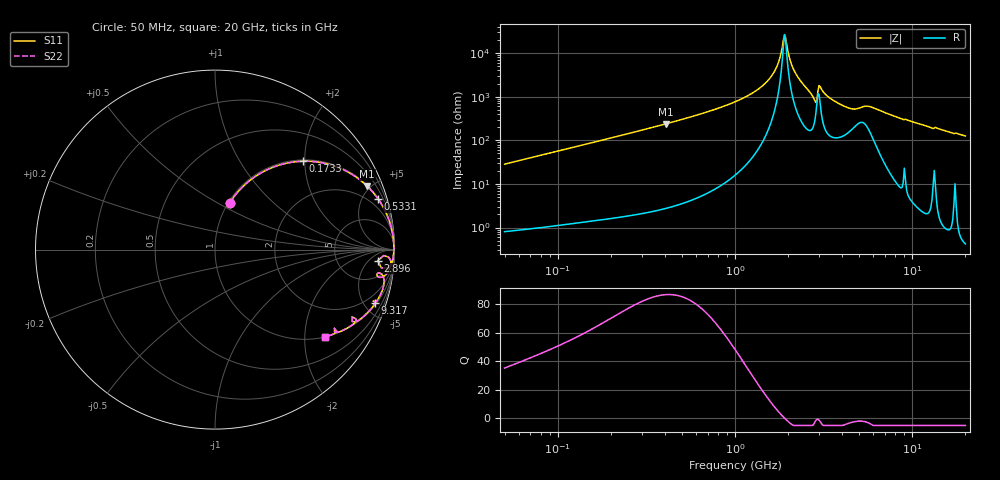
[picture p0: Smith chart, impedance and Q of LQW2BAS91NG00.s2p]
!Murata Part Number: LQW2BAS91NG00
!These Parameters are Measured in Series Mode Connection
!  o--[Z]--o
!Port1  Port2
!  o-------o
!Freq. Start=50[MHz] Stop=20[GHz], 401[Steps]
# Hz S RI R 50
!Freq.(Hz) S11(Real) S11(Imag) S21(Real) S21(Imag) S12(Real) S12(Imag) S22(Real) S22(Imag)
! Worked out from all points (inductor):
!   401 points, 50 MHz to 20 GHz, reference 50 ohm
!   read as one part in series: L = 90.2 nH near 51.52 MHz
!   highest Q = 86.9 at 407.1 MHz (marker M1), where L = 93.3 nH
!   self-resonance near 1.904 GHz
!   S11 on the Smith chart (normalised r, x): 50 MHz: 1.02, +0.57; 173.3 MHz: 1.03, +1.97; 533.1 MHz: 1.08, +6.46; 2.896 GHz: 14, -10; 9.317 GHz: 1.14, -5.91; 20 GHz: 1.01, -2.52
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5e7  0.081 0.2591  0.919 -0.2591  0.919 -0.2591  0.081 0.2591
1.364002e8  0.3756 0.4759  0.6244 -0.4759  0.6244 -0.4759  0.3756 0.4759
1.733395e8  0.4915 0.4924  0.5085 -0.4924  0.5085 -0.4924  0.4915 0.4924
3.721004e8  0.8214 0.3773  0.1786 -0.3773  0.1786 -0.3773  0.8214 0.3773
4.070905e8  0.8478 0.3535  0.1522 -0.3535  0.1522 -0.3535  0.8478 0.3535
5.330693e8  0.9098 0.2806  0.0902 -0.2806  0.0902 -0.2806  0.9098 0.2806
1e9  0.9806 0.1281  0.0194 -0.1281  0.0194 -0.1281  0.9806 0.1281
1.309461e9  0.9919 0.0728  0.00814 -0.0728  0.00814 -0.0728  0.9919 0.0728
1.567309e9  0.9955 0.038  0.00451 -0.038  0.00451 -0.038  0.9955 0.038
1.740566e9  0.9963 0.0179  0.00366 -0.0179  0.00366 -0.0179  0.9963 0.0179
1.904239e9  0.9963 0.000534  0.00369 -0.000534  0.00369 -0.000534  0.9963 0.000534
2.179053e9  0.9947 -0.0265  0.00529 0.0265  0.00529 0.0265  0.9947 -0.0265
2.728004e9  0.9764 -0.0887  0.0236 0.0887  0.0236 0.0887  0.9764 -0.0887
2.810964e9  0.9538 -0.1041  0.0462 0.1041  0.0462 0.1041  0.9538 -0.1041
2.896447e9  0.9078 -0.0609  0.0922 0.0609  0.0922 0.0609  0.9078 -0.0609
3.029571e9  0.9746 -0.0519  0.0254 0.0519  0.0254 0.0519  0.9746 -0.0519
3.415248e9  0.9753 -0.101  0.0247 0.101  0.0247 0.101  0.9753 -0.101
4.212059e9  0.9382 -0.1499  0.0618 0.1499  0.0618 0.1499  0.9382 -0.1499
5.598765e9  0.9288 -0.1376  0.0712 0.1376  0.0712 0.1376  0.9288 -0.1376
7.442007e9  0.9298 -0.233  0.0702 0.233  0.0702 0.233  0.9298 -0.233
9.316812e9  0.8917 -0.2989  0.1083 0.2989  0.1083 0.2989  0.8917 -0.2989
2e10  0.6127 -0.4855  0.3873 0.4855  0.3873 0.4855  0.6127 -0.4855
